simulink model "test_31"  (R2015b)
settings: Solver=FixedStepDiscrete  StartTime=0.0  StopTime=200.0  RelTol=1e-3
undefined symbols (not defined in the file or in its folder): fir1
libraries: simulink x1, dspsigops x1, dspstat3 x1

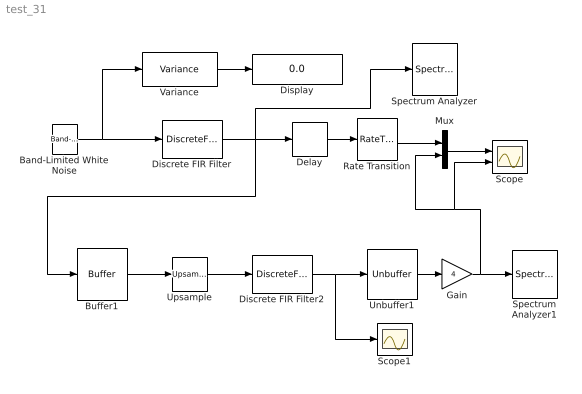
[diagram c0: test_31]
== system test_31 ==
  Band-Limited White Noise : simulink/Sources/Band-Limited White Noise  Cov=[0.01]  Ts=0.01  seed=[23341]
  Buffer1 : Buffer  N=2048  TreatMby1Signals=One channel  OutputFrames=off
  Delay : Delay  DelayLength=2*2048+512+32-1  InputProcessing=Inherited
  Discrete FIR Filter : DiscreteFir  Coefficients=fir1(256, 0.25);
  Discrete FIR Filter2 : DiscreteFir  Coefficients=fir1(256, 0.25);  InputProcessing=Columns as channels (frame based)
  Display : Display
  Gain : Gain  Gain=4
  Mux : Mux  Inputs=2
  Rate Transition : RateTransition
  Scope : Scope  NumInputPorts=2
  Scope1 : Scope
  Spectrum Analyzer : SpectrumAnalyzer
  Spectrum Analyzer1 : SpectrumAnalyzer
  Unbuffer1 : Unbuffer  SampleBasedProcessing=Same as frame based
  Upsample : dspsigops/Upsample  N=4  phase=0  InputProcessing=Columns as channels (frame based)  RateOptions=Allow multirate processing  ic=0  mode=Unused parameter value
  Variance : dspstat3/Variance  run=on  reset_popup=None  directionMode=Each column  dimension=1  roiEnable=off  roiType=Rectangles  roiPortion=Entire ROI  roiOutput=Individual statistics for each ROI  roiFlag=off  roundingMode=Floor  overflowMode=off
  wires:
  Band-Limited White Noise/1 -> Variance/1, Discrete FIR Filter/1
  Mux/1 -> Scope/1
  Discrete FIR Filter/1 -> Buffer1/1, Delay/1, Spectrum Analyzer/1
  Variance/1 -> Display/1
  Buffer1/1 -> Upsample/1
  Discrete FIR Filter2/1 -> Scope1/1, Unbuffer1/1
  Unbuffer1/1 -> Gain/1
  Upsample/1 -> Discrete FIR Filter2/1
  Delay/1 -> Rate Transition/1
  Gain/1 -> Mux/2, Scope/2, Spectrum Analyzer1/1
  Rate Transition/1 -> Mux/1
